(* Logix 5000 AddOnInstructionDefinition export AMCI_5034_PTO_AM_Run_Blend; software revision 37.00 *)

TYPE AMCI_5034_PTO_AM_Input_Data :
STRUCT
   ConnectionFaulted : DINT;
   MovingCW : BOOL;
   MovingCCW : BOOL;
   InHoldState : BOOL;
   Stopped : BOOL;
   AtHome : BOOL;
   Accelerating : BOOL;
   Decelerating : BOOL;
   MoveComplete : BOOL;
   HomeInvalid : BOOL;
   InvalidProfile : BOOL;
   PositionInvalid : BOOL;
   InputError : BOOL;
   CommandError : BOOL;
   ConfigurationError : BOOL;
   ModuleOK : BOOL;
   GeneralPurposeOutputStatus : BOOL;
   Input1Active : BOOL;
   Input2Active : BOOL;
   Input3Active : BOOL;
   Input4Active : BOOL;
   bit_20_reserved : BOOL;
   bit_21_reserved : BOOL;
   bit_22_reserved : BOOL;
   EncoderFollowerMode : BOOL;
   BlendMoveRunning : BOOL;
   BlendMoveAcknowledge : BOOL;
   MinimumRegistrationProgrammed : BOOL;
   EncoderMotionDirection : BOOL;
   MultipleInputsWithSameFunction : BOOL;
   FSCExceedsNumberOfDataBits : BOOL;
   AbsoluteEncoderSetupError : BOOL;
   bit_31_reserved : BOOL;
   CurrentPosition : DINT;
   EncoderPosition : DINT;
   CapturedPosition : DINT;
END_STRUCT
END_TYPE

TYPE AMCI_5034_PTO_AM_Output_Data :
STRUCT
   Command_Word : DINT;
   TargetPosition : DINT;
   TargetVelocity : UDINT;
   Acceleration : DINT;
   Deceleration : DINT;
END_STRUCT
END_TYPE

ADD_ON_INSTRUCTION AMCI_5034_PTO_AM_Run_Blend   (* revision 1.0, vendor AMCI, ExecuteEnableInFalse *)
// Revision note:
// 10/01/2025 initial release
// Help:
// AXIS INPUT DATA:  Input data from the AMCI 5034-PTO-AM.   Uses the AMCI_5034_PTO_Input_Data User Defined Data Type.
// AXIS OUTPUT DATA; Output data from the AOI to the AMCI 5034-PTO-AM.    Uses the AMCI_5034_PTO_Output_Data User Defined Data Type.
// DIRECTION_0_POSITIVECW_1_NEGATIVECCW: Selects the direction in which the Blend Move will be run.
// EN (Enable) Set when rung is true, Reset when rung is false
// DN (Done) Set when command is sent to the motion device.  Reset when the rung is false.
// ER (Error) Set when a command, input, configuraiton, or profile error.   Reset when the rung is false.
VAR_IN_OUT
   Axis_Input_Data : AMCI_5034_PTO_AM_Input_Data; {required}
   Axis_Output_Data : AMCI_5034_PTO_AM_Output_Data; {required}
END_VAR
VAR_INPUT
   Direction_0_PositiveCW_1_NegativeCCW : BOOL; {required}
END_VAR
VAR_OUTPUT
   EN : BOOL; {visible}   // set when rung with AOI is true and the Move Complete stetus bit is off.
   DN : BOOL; {access Read Only, visible}   // set when preset motor position command sent to motion axis
   ER : BOOL; {access Read Only, visible}   // set when input, command, or configuraiton error
END_VAR
VAR
   command_data_block : DINT[5];
        [0]   // Command Bits MSW
        [1]   // Target Position
        [2]   // Upper Target Position
        [3]   // Lower Target Position
        [4]   // Upper Programmed Speed
END_VAR

ROUTINE EnableInFalse   (* ladder *)
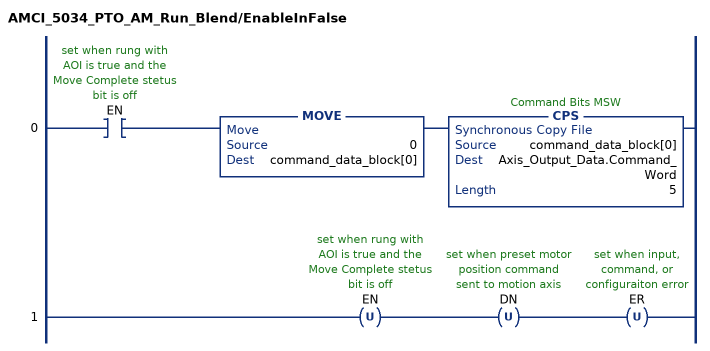
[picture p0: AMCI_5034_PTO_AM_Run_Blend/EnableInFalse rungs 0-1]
   0: XIC(EN)MOVE(0,command_data_block[0])CPS(command_data_block[0],Axis_Output_Data.Command_Word,5);
   1: OTU(EN)OTU(DN)OTU(ER);
END_ROUTINE

ROUTINE Logic   (* ladder *)
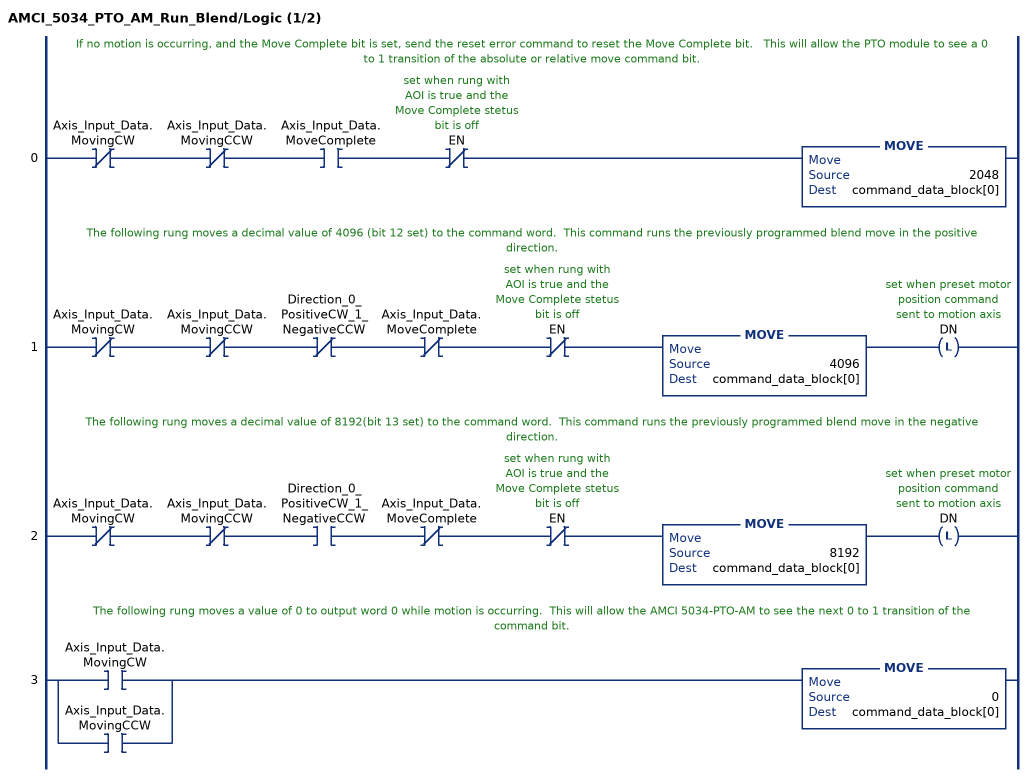
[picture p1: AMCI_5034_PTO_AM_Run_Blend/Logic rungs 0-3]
   // If no motion is occurring, and the Move Complete bit is set, send the reset error command to reset the Move Complete bit.   This will allow the PTO module to see a 0 to 1 transition of the absolute or relative move command bit.
   0: XIO(Axis_Input_Data.MovingCW)XIO(Axis_Input_Data.MovingCCW)XIC(Axis_Input_Data.MoveComplete)XIO(EN)MOVE(2048,command_data_block[0]);
   // The following rung moves a decimal value of 4096 (bit 12 set) to the command word.  This command runs the previously programmed blend move in the positive direction.
   1: XIO(Axis_Input_Data.MovingCW)XIO(Axis_Input_Data.MovingCCW)XIO(Direction_0_PositiveCW_1_NegativeCCW)XIO(Axis_Input_Data.MoveComplete)XIO(EN)MOVE(4096,command_data_block[0])OTL(DN);
   // The following rung moves a decimal value of 8192(bit 13 set) to the command word.  This command runs the previously programmed blend move in the negative direction.
   2: XIO(Axis_Input_Data.MovingCW)XIO(Axis_Input_Data.MovingCCW)XIC(Direction_0_PositiveCW_1_NegativeCCW)XIO(Axis_Input_Data.MoveComplete)XIO(EN)MOVE(8192,command_data_block[0])OTL(DN);
   // The following rung moves a value of 0 to output word 0 while motion is occurring.  This will allow the AMCI 5034-PTO-AM to see the next 0 to 1 transition of the command bit.
   3: [XIC(Axis_Input_Data.MovingCW) ,XIC(Axis_Input_Data.MovingCCW) ]MOVE(0,command_data_block[0]);
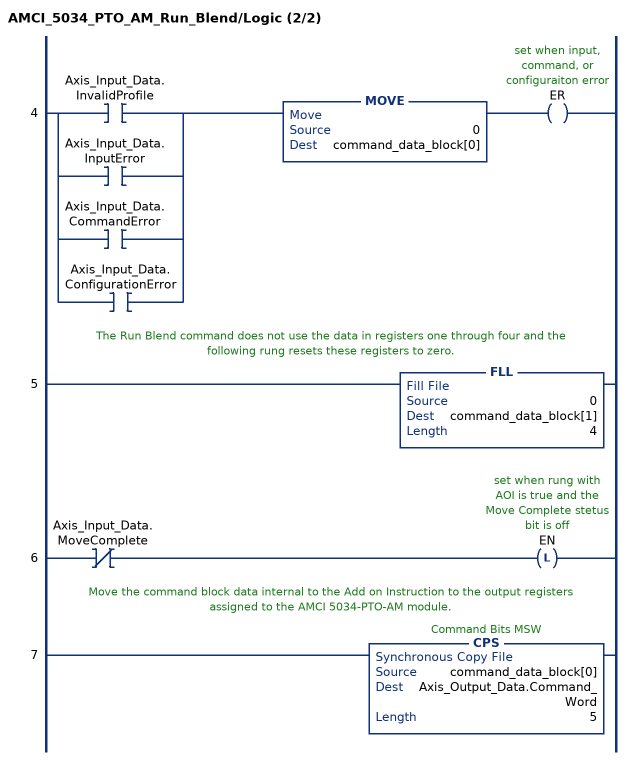
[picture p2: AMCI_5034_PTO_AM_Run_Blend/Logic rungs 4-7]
   4: [XIC(Axis_Input_Data.InvalidProfile) ,XIC(Axis_Input_Data.InputError) ,XIC(Axis_Input_Data.CommandError) ,XIC(Axis_Input_Data.ConfigurationError) ]MOVE(0,command_data_block[0])OTE(ER);
   // The Run Blend command does not use the data in registers one through four and the following rung resets these registers to zero.
   5: FLL(0,command_data_block[1],4);
   6: XIO(Axis_Input_Data.MoveComplete)OTL(EN);
   // Move the command block data internal to the Add on Instruction to the output registers assigned to the AMCI 5034-PTO-AM module.
   7: CPS(command_data_block[0],Axis_Output_Data.Command_Word,5);
END_ROUTINE
END_ADD_ON_INSTRUCTION
